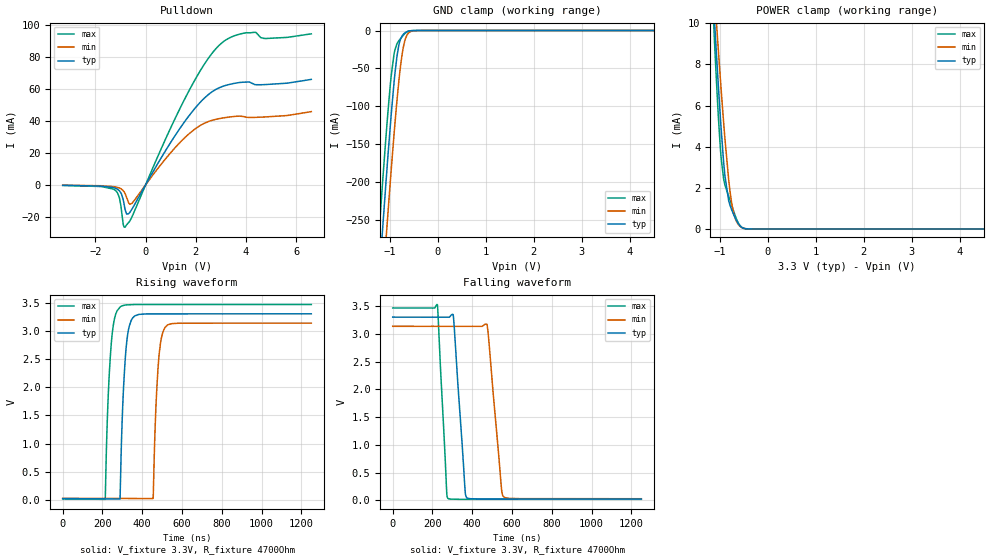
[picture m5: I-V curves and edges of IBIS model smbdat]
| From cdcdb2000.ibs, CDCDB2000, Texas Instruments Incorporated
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[Model]   smbdat
Model_type   I/O_open_drain
Polarity   Inverting
Enable   Active-High
Vinl = 0.6
Vinh = 1.2
Vmeas = 1.65
Vref = 3.3
Cref = 2pF
Rref = 4700
|   typ   min   max
C_comp   2.397pF   2.310pF   2.475pF
|  Where Nom  PVT is Nominal Process, 3.3V,   32C
|   Fast PVT is Strong Process,  3.465, -35C
|   Slow PVT is Weak Process,   3.135V, 110C
[Voltage Range]   3.3   3.135   3.465
|Junction Temperature
[Temperature Range]   32   110   -35
[Pullup Reference]   3.3   3.135   3.465
[Pulldown Reference]   0   0   0
[Power Clamp Reference]   3.3   3.135   3.465
[GND Clamp Reference]   0   0   0
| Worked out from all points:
|   slope of the pulldown table from 0 to 0.495 V, typ, clamps not added: 36.5 ohm
|   GND clamp passes 1 mA (typ) near -0.62 V on its own axis
|   POWER clamp passes 1 mA (typ) near -0.76 V on its own axis
|   falling waveform, V_fixture 3.3V, R_fixture 4700Ohm: 20-80 % time 37.2ns typ, 45ns min, 29.2ns max; typ from 3.3 V to 0.025 V
|   rising waveform, V_fixture 3.3V, R_fixture 4700Ohm: 20-80 % time 24.8ns typ, 23.8ns min, 25.9ns max; typ from 0.025 V to 3.3 V
[Pulldown]
|   Voltage   I(typ)   I(min)   I(max)
-3.3V     -272.1uA   -202.9uA   -338.3uA
-1.241V   -1.867mA   -1.167mA   -2.984mA
-1.053V   -3.524mA   -1.892mA   -7.513mA
-894.3mV  -9.033mA   -3.544mA   -24.26mA
-815.1mV  -15.57mA   -5.476mA   -26.4mA
-755.7mV  -18.25mA   -7.828mA   -24.93mA
-547.8mV  -15.28mA   -11.61mA   -20.21mA
1.541V    39.15mA    29.16mA    53.09mA
2.927V    60.61mA    41.37mA    87.13mA
4.036V    64.21mA    42.21mA    95.01mA
4.788V    62.66mA    42.45mA    91.41mA
6.6V      65.87mA    45.75mA    94.33mA
[GND Clamp]
|   Voltage   I(typ)   I(min)   I(max)
-3.3V     -2.34A     -2.409A    -2.285A
-1.231V   -332.9mA   -409.9mA   -270.6mA
-1.142V   -252.8mA   -329.5mA   -191.2mA
-1.082V   -200.9mA   -277.1mA   -140.8mA
-1.053V   -175.7mA   -251.4mA   -116.8mA
-973.5mV  -111.7mA   -184.7mA   -60.4mA
-914.1mV  -69.11mA   -137.4mA   -31.5mA
-854.7mV  -35.1mA    -93.91mA   -17.79mA
-745.8mV  -7.175mA   -31.85mA   -8.177mA
-646.8mV  -1.607mA   -6.523mA   -1.956mA
-399.3mV  -3.704uA   -33.43uA   -672.6nA
6.6V      0A         0A         0A
[POWER Clamp]
|   Voltage   I(typ)   I(min)   I(max)
-3.3V     110.9mA    95.66mA    136.2mA
-1.221V   14.71mA    15.34mA    14.77mA
-1.112V   10.13mA    11.45mA    9.124mA
-1.082V   8.931mA    10.42mA    7.695mA
-1.043V   7.379mA    9.067mA    5.921mA
-983.4mV  5.202mA    7.1mA      3.739mA
-894.3mV  2.571mA    4.378mA    2.131mA
-795.3mV  1.202mA    1.961mA    1.448mA
-726mV    772.5uA    911.6uA    955.4uA
-636.9mV  340uA      294.9uA    394.9uA
-508.2mV  39.45uA    35.79uA    30.99uA
6.6V      0A         0A         0A
[Ramp]
R_load = 4700
|   typ   min   max
dV/dt_r   1.96506/2.47825e-08   1.86267/2.38452e-08   2.06717/2.58911e-08
dV/dt_f   1.96506/3.72334e-08   1.86266/4.49653e-08   2.06717/2.91867e-08
[Falling Waveform]
V_fixture = 3.3V
V_fixture_min = 3.135V
V_fixture_max = 3.465V
R_fixture = 4700Ohm
C_fixture = 0F
|   Time   V(typ)   V(min)   V(max)
0s        3.3V       3.135V     3.465V
224.7ns   3.299V     3.135V     3.524V
278ns     3.299V     3.134V     35.89mV
305ns     3.317V     3.134V     22.23mV
364ns     173.6mV    3.134V     20.2mV
373.3ns   46.63mV    3.134V     20.2mV
474.7ns   25.82mV    3.156V     20.14mV
546.8ns   25.73mV    213.9mV    20.1mV
560.6ns   25.72mV    57.57mV    20.09mV
1.25us    24.84mV    30.47mV    19.68mV
[Rising Waveform]
V_fixture = 3.3V
V_fixture_min = 3.135V
V_fixture_max = 3.465V
R_fixture = 4700Ohm
C_fixture = 0F
|   Time   V(typ)   V(min)   V(max)
0s        24.84mV    30.47mV    19.68mV
213.6ns   20.48mV    28.44mV    12.36mV
243ns     19.88mV    28.16mV    2.719V
289.3ns   161.1mV    27.72mV    3.423V
316.4ns   2.595V     27.46mV    3.457V
360.2ns   3.257V     27.04mV    3.464V
454.8ns   3.299V     38.1mV     3.464V
482.7ns   3.299V     2.494V     3.464V
525.1ns   3.299V     3.095V     3.464V
1.25us    3.3V       3.135V     3.465V
